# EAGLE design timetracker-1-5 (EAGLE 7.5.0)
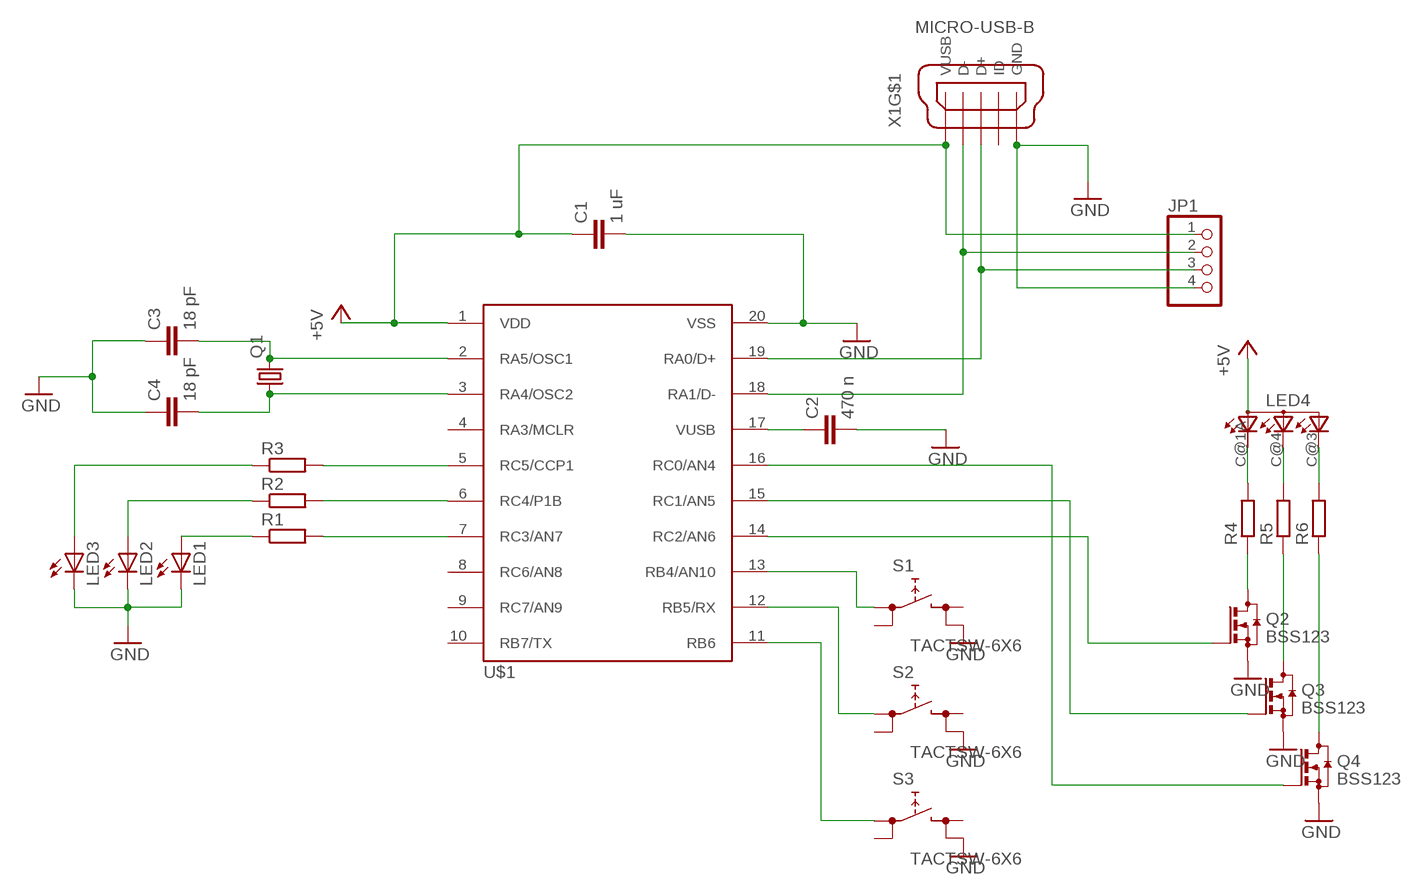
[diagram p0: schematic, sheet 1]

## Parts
C1  1 uF  C-EUC0805  [C0805]
C2  470 n  C-EUC0805  [C0805]
C3  18 pF  C-EUC0805  [C0805]
C4  18 pF  C-EUC0805  [C0805]
JP1  PINHD-1X4  [1X04]
LED1  LEDSML0805  [SML0805]
LED2  LEDSML0805  [SML0805]
LED3  LEDSML0805  [SML0805]
LED4  RGBLED-3P-LCC-4  [P-LCC-4]
Q1  CRYSTALHC49UP  [HC49UP]
Q2  BSS123  [SOT23]
Q3  BSS123  [SOT23]
Q4  BSS123  [SOT23]
R1  R-EU_R0805  [R0805]
R2  R-EU_R0805  [R0805]
R3  R-EU_R0805  [R0805]
R4  R-EU_R0805  [R0805]
R5  R-EU_R0805  [R0805]
R6  R-EU_R0805  [R0805]
S1  TACTSW-6X6  [TACTSW-6X6]
S2  TACTSW-6X6  [TACTSW-6X6]
S3  TACTSW-6X6  [TACTSW-6X6]
U$1  PIC18F14K50SMD  [DIL20-SMD]
X1  MICRO-USB-B  [MICRO-B-PAC]

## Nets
+5V: C1.1 JP1.1 LED4.A(A2) U$1.1(VDD) X1.1(VUSB)
GND: C1.2 C2.2 C3.1 C4.1 JP1.4 LED1.C LED2.C LED3.C Q2.2(S) Q3.2(S) Q4.2(S) S1.4(2.2) S2.4(2.2) S3.4(2.2) U$1.20(VSS) X1.5(GND)
N$1: C2.1 U$1.17(VUSB)
N$2: C3.2 Q1.2 U$1.2(RA5/OSC1)
N$3: C4.2 Q1.1 U$1.3(RA4/OSC2)
N$4: JP1.3 U$1.19(RA0/D+) X1.3(D+)
N$5: JP1.2 U$1.18(RA1/D-) X1.2(D-)
N$8: LED1.A R1.1
N$9: R1.2 U$1.7(RC3/AN7)
N$10: R2.2 U$1.6(RC4/P1B)
N$11: LED2.A R2.1
N$12: R3.2 U$1.5(RC5/CCP1)
N$13: LED3.A R3.1
N$14: Q2.3(D) R4.1
N$15: LED4.C@1(CRED) R4.2
N$16: Q2.1(G) U$1.14(RC2/AN6)
N$17: Q3.1(G) U$1.15(RC1/AN5)
N$18: Q4.1(G) U$1.16(RC0/AN4)
N$19: LED4.C@4(CGREEN) R5.2
N$20: LED4.C@3(CBLUE) R6.2
N$21: Q3.3(D) R5.1
N$22: Q4.3(D) R6.1
N$23: S1.1(1.1) U$1.13(RB4/AN10)
N$24: S2.1(1.1) U$1.12(RB5/RX)
N$25: S3.1(1.1) U$1.11(RB6)
Unconnected: S1.2(1.2) S1.3(2.1) S2.2(1.2) S2.3(2.1) S3.2(1.2) S3.3(2.1) U$1.4(RA3/MCLR) U$1.8(RC6/AN8) U$1.9(RC7/AN9) U$1.10(RB7/TX) X1.4(ID) X1.M1(S:S1) X1.M2(S:S2) X1.M3(S:S3) X1.M4(S:S4)

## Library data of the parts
C1-C4 = rcl:C-EU: CAPACITOR, European symbol
JP1 = pinhead:PINHD-1X4: PIN HEADER
LED1-LED3 = led:LED: LED
LED4 = g-e2e-training:RGBLED-3: OSRAM - Hyper Multi TOPLED® (RGB) LB E673, LV E673, LT E673 - Power TOPLED® Enhanced optical Power LED (HOP2000) LS E67B, LA E67B, LO E67B, LY E67B - Hyper Multi TOPLED® Enhanced optical Power LED (HOP2000 / ATON®) LATB T66B - Hyper Multi TOPLED® Hyper-Bright LED LATB T686 Source: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
Q1 = crystal:CRYSTAL: CRYSTAL; OC_FARNELL: unknown; OC_NEWARK: unknown
Q2-Q4 = transistor-small-signal:BSS123: N-CHANNEL MOS FET
R1-R6 = rcl:R-EU_: RESISTOR, European symbol
S1-S3 = g-e2e-training:TACTSW-6X6: 6.2 X 6.5mm TACT Switch (SMD) Source: http://www3.alps.co.jp/WebObjects/catalog.woa/PDF/E/Switch/Tact/SKHM/SKHM.PDF
U$1 = timetracker:PIC18F14K50
X1 = g-e2e-training:MICRO-USB-B: MINI USB-B Conector Source: www.cypressindustries.com

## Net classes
0 default: width 0.305 mm

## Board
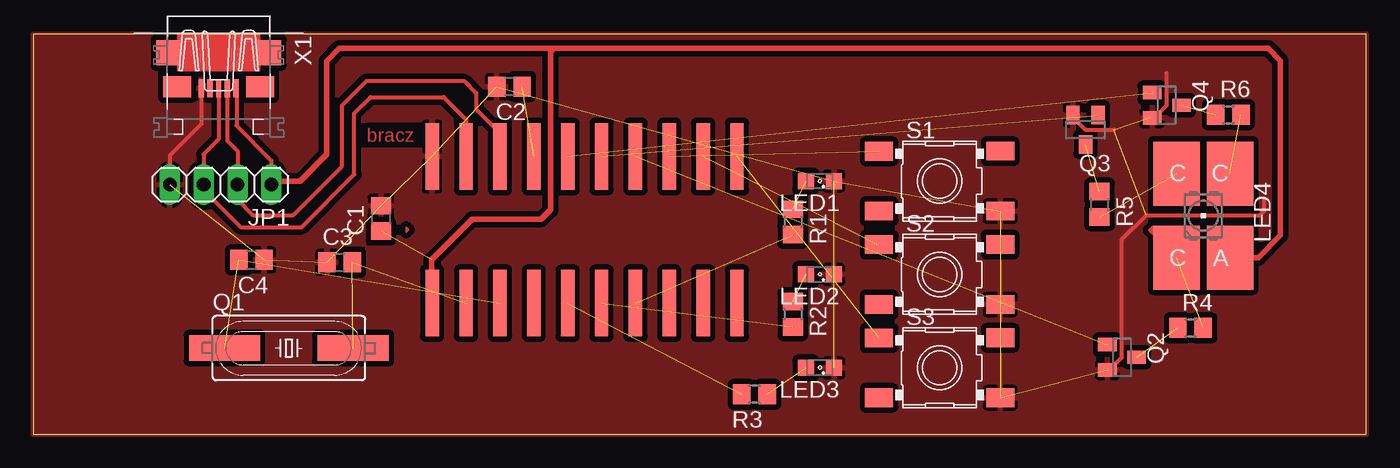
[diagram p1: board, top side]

Size 100 x 30 mm. Coordinates in mm from the lower left corner, seen from the top.
Outline: 0,0 100,0 100,30 0,30 0,0
Copper layers (1*16): Top 0.035mm / dielectric 1.5mm / Bottom 0.035mm
Design rules "default *": minimum track width 10mil, minimum drill 24mil, track to track 16mil, track to pad 16mil, pad to pad 8mil, via to via 8mil, smd to smd 8mil, copper to edge 0mil, drill to drill 8mil, minimum pad ring 10mil, minimum via ring 8mil, stop-mask expansion 4mil, vias tented up to drill 0mil, thermal gap 10mil

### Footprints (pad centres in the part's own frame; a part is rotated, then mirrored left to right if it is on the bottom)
C0805 = smd 1.3 x 1.5: 1 -0.95,0; 2 0.95,0
1X04 = drill 1.016 long: 1 -3.81,0; 2 -1.27,0; 3 1.27,0; 4 3.81,0
SML0805 = smd 1.2 x 1.2: A 1.05,0; C -1.05,0
P-LCC-4 = smd 3.5 x 4.8: A -2,3.15; C@1 2,3.15; C@3 -2,-3.15; C@4 2,-3.15
HC49UP = smd 5.334 x 1.93: 1 -4.826,0; 2 4.826,0
SOT23 = smd 1 x 1.4: 1 -0.95,-1.1; 2 0.95,-1.1; 3 0,1.1
R0805 = smd 1.3 x 1.5: 1 -0.95,0; 2 0.95,0
TACTSW-6X6 = smd 2.1 x 1.4: 1 -4.55,2.24; 2 4.55,2.25; 3 -4.55,-2.25; 4 4.55,-2.25
DIL20-SMD = smd 1 x 5: 1 -11.43,-5.5; 2 -8.89,-5.5; 3 -6.35,-5.5; 4 -3.81,-5.5; 5 -1.27,-5.5; 6 1.27,-5.5; 7 3.81,-5.5; 8 6.35,-5.5; 9 8.89,-5.5; 10 11.43,-5.5; 11 11.43,5.5; 12 8.89,5.5; 13 6.35,5.5; 14 3.81,5.5; 15 1.27,5.5; 16 -1.27,5.5; 17 -3.81,5.5; 18 -6.35,5.5; 19 -8.89,5.5; 20 -11.43,5.5
MICRO-B-PAC = smd 1.35 x 0.4: 1 2.675,1.3; 2 2.675,0.65; 3 2.675,0; 4 2.675,-0.65; 5 2.675,-1.3 | smd 1.9 x 1.8: M1 0,-3.8; M2 0,3.8 | smd 1.6 x 2.1: M3 2.55,3.1; M4 2.55,-3.1

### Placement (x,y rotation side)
C1  26.09,16.2 90 top
C2  35.72,26.09 180 top
C3  22.98,12.91 0 top
C4  16.37,13.09 180 top
JP1  14.05,18.74 180 top
LED1  59,19 180 top
LED2  59,12 180 top
LED3  59,5 180 top
LED4  87.78,16.41 180 top
Q1  19.17,6.48 0 top
Q2  81.69,5.79 270 top
Q3  78.94,22.86 180 top
Q4  85.04,24.69 270 top
R1  56.99,15.94 270 top
R2  56.99,9.02 270 top
R3  54.1,3.01 180 top
R4  86.82,7.99 0 top
R5  79.99,17.26 270 top
R6  89.66,23.99 0 top
S1  68,19 0 top
S2  68,12 0 top
S3  68,5 0 top
U$1  41.36,15.35 0 top
X1  13.9,28.64 270 top

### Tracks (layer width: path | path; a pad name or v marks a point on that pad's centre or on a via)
+5V  (1 unrouted)
  Top 0.305: X1.1 15.24,25.93 15.24,23.16 17.86,20.55 JP1.1
  Top 0.406: JP1.1 18.12,19 20,19 22,21 22,28 22.96,28.96 39.01,28.96 | 39.01,28.96 92.66,28.96 93.57,28.04 93.57,14.94 91.9,13.26 LED4.A | U$1.1 29.87,9.91 29.87,13.11 32.92,16.15 38.1,16.15 38.81,16.87 38.81,28.75 39.01,28.96
GND  (14 unrouted)
  Top 0.305: Q3.2 77.99,23.81 78.94,22.86 81.08,22.86 | Q4.2 83.86,23.74 83.82,23.77 84.12,23.77 85.04,24.69 85.04,27.13 | Q2.2 80.74,4.84 81.69,5.79 81.69,14.63 83.52,16.46 92.05,16.46 92.35,16.76 92.35,17.68 | X1.5 12.61,23.27 10.24,20.91 JP1.4
  pour Top (isolate 0.356): 0,30 0,0 100,0 100,30
N$1  (1 unrouted)
N$2  (2 unrouted)
N$3  (2 unrouted)
N$4
  Top 0.305: U$1.19 32.47,23.61 30.79,25.3 25.3,25.3 24.08,24.08 24.08,19.51 20.12,15.54 15.54,15.54 12.78,18.31 JP1.3 12.78,21.01 13.9,22.14 X1.3
N$5
  Top 0.305: U$1.18 35.01,22.6 33.22,24.38 33.22,25.6 32.31,26.52 24.99,26.52 23.16,24.69 23.16,20.12 19.51,16.46 16.46,16.46 15.32,17.6 JP1.2 15.32,21.26 14.55,22.02 X1.2
N$8  (1 unrouted)
N$9  (1 unrouted)
N$10  (1 unrouted)
N$11  (1 unrouted)
N$12  (1 unrouted)
N$13  (1 unrouted)
N$14  (1 unrouted)
N$15  (1 unrouted)
N$16  (1 unrouted)
N$17  (1 unrouted)
N$18  (1 unrouted)
N$19  (1 unrouted)
N$20  (1 unrouted)
N$21  (1 unrouted)
N$22  (1 unrouted)
N$23  (1 unrouted)
N$24  (1 unrouted)
N$25  (1 unrouted)

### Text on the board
Top: bracz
